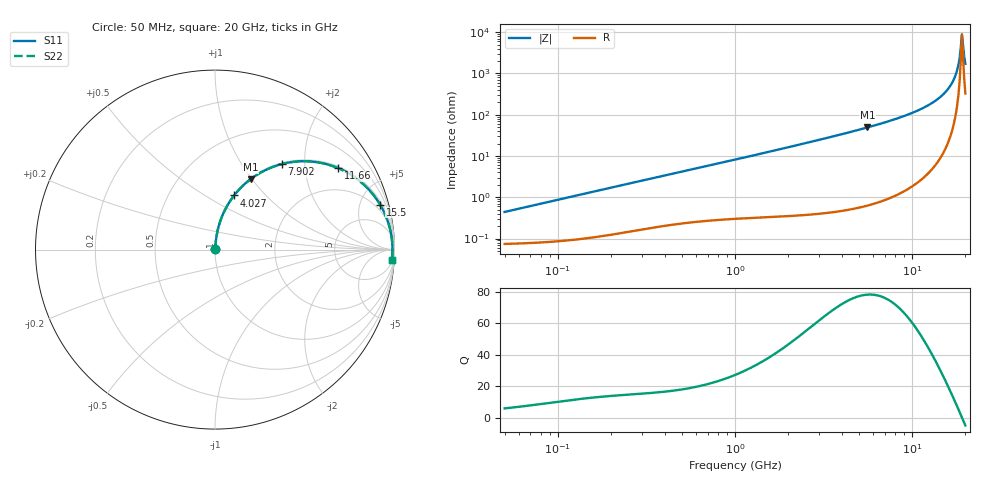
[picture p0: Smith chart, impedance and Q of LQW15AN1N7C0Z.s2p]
!Murata Part Number: LQW15AN1N7C0Z
!These Parameters are Measured in Series Mode Connection
!  o--[Z]--o
!Port1  Port2
!  o-------o
!Freq. Start=50[MHz] Stop=20[GHz], 401[Steps]
# Hz S RI R 50
!Freq.(Hz) S11(Real) S11(Imag) S21(Real) S21(Imag) S12(Real) S12(Imag) S22(Real) S22(Imag)
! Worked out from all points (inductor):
!   401 points, 50 MHz to 20 GHz, reference 50 ohm
!   read as one part in series: L = 1.38 nH near 51.52 MHz
!   highest Q = 78.4 at 5.599 GHz (marker M1), where L = 1.4 nH
!   self-resonance near 19.12 GHz
!   S11 on the Smith chart (normalised r, x): 50 MHz: 1.00, +0.01; 4.027 GHz: 1.01, +0.68; 7.902 GHz: 1.02, +1.53; 11.66 GHz: 1.06, +2.99; 15.5 GHz: 1.32, +7.25; 20 GHz: 8, -34
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5e7  0.000759 0.00434  0.9992 -0.00434  0.9992 -0.00434  0.000759 0.00434
1.364002e8  0.00112 0.0118  0.9989 -0.0118  0.9989 -0.0118  0.00112 0.0118
3.721004e8  0.0029 0.0311  0.9971 -0.0311  0.9971 -0.0311  0.0029 0.0311
1e9  0.00954 0.0805  0.9905 -0.0805  0.9905 -0.0805  0.00954 0.0805
2.728004e9  0.0512 0.2121  0.9488 -0.2121  0.9488 -0.2121  0.0512 0.2121
4.026975e9  0.1066 0.3017  0.8934 -0.3017  0.8934 -0.3017  0.1066 0.3017
5.598765e9  0.1985 0.3925  0.8015 -0.3925  0.8015 -0.3925  0.1985 0.3925
7.442007e9  0.3345 0.4652  0.6655 -0.4652  0.6655 -0.4652  0.3345 0.4652
7.901521e9  0.3719 0.4765  0.6281 -0.4765  0.6281 -0.4765  0.3719 0.4765
9.745021e9  0.5281 0.4912  0.4719 -0.4912  0.4719 -0.4912  0.5281 0.4912
1.166392e10  0.6868 0.4537  0.3132 -0.4537  0.3132 -0.4537  0.6868 0.4537
1.375312e10  0.8326 0.3592  0.1674 -0.3592  0.1674 -0.3592  0.8326 0.3592
1.550395e10  0.92 0.2504  0.08 -0.2504  0.08 -0.2504  0.92 0.2504
1.670968e10  0.9592 0.1676  0.0408 -0.1676  0.0408 -0.1676  0.9592 0.1676
1.747767e10  0.9753 0.1138  0.0247 -0.1138  0.0247 -0.1138  0.9753 0.1138
1.800918e10  0.9827 0.0767  0.0173 -0.0767  0.0173 -0.0767  0.9827 0.0767
1.855685e10  0.9872 0.0391  0.0128 -0.0391  0.0128 -0.0391  0.9872 0.0391
1.88369e10  0.9884 0.0201  0.0116 -0.0201  0.0116 -0.0201  0.9884 0.0201
1.912117e10  0.9888 0.0011  0.0112 -0.0011  0.0112 -0.0011  0.9888 0.0011
1.940974e10  0.9886 -0.0179  0.0114 0.0179  0.0114 0.0179  0.9886 -0.0179
1.970266e10  0.9875 -0.0369  0.0125 0.0369  0.0125 0.0369  0.9875 -0.0369
2e10  0.9858 -0.0558  0.0142 0.0558  0.0142 0.0558  0.9858 -0.0558
